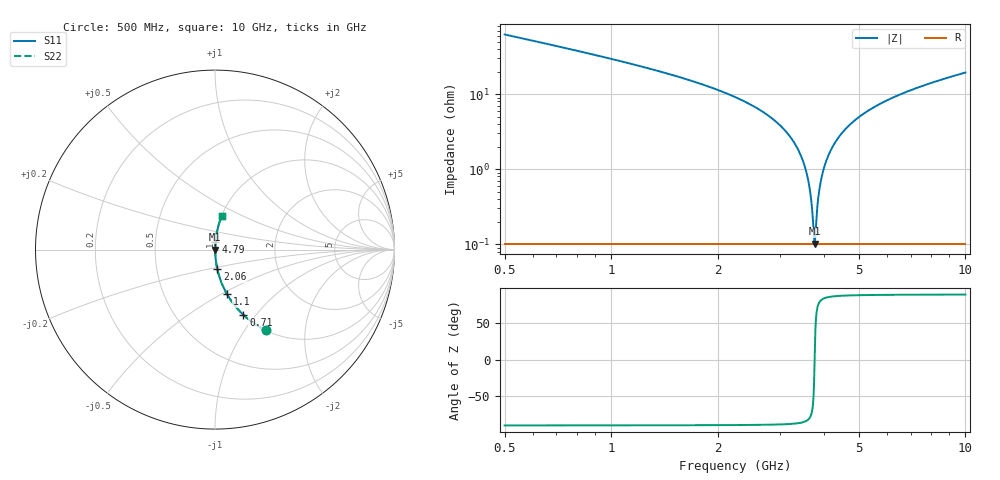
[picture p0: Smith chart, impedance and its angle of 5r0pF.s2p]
! Created Fri Jan 10 15:51:09 2014
# hz S db R 50
! 2 Port Network Data from SP1.SP block
! freq  dbS11  angS11  dbS21  angS21  dbS12  angS12  dbS22  angS22
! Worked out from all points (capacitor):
!   951 points, 500 MHz to 10 GHz, reference 50 ohm
!   read as one part in series: C = 5 pF near 540 MHz
!   lowest |Z| = 101 mohm at 3.75 GHz (marker M1)
!   series resonance near 3.752 GHz, so ESL is about 360 pH
!   S11 on the Smith chart (normalised r, x): 500 MHz: 1.00, -1.25; 710 MHz: 1.00, -0.86; 1.1 GHz: 1.00, -0.53; 2.06 GHz: 1.00, -0.22; 4.79 GHz: 1.00, +0.08; 10 GHz: 1.00, +0.39
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5e8  -5.52 -57.9  -1.44 32.0  -1.44 32.0  -5.52 -57.9
7.1e8  -8.04 -66.5  -0.75 23.4  -0.75 23.4  -8.04 -66.5
1.1e9  -11.85 -75.0  -0.30 14.8  -0.30 14.8  -11.85 -75.0
2.06e9  -19.40 -83.3  -0.06 6.2  -0.06 6.2  -19.40 -83.3
2.09e9  -19.63 -83.5  -0.06 6.0  -0.06 6.0  -19.63 -83.5
2.79e9  -25.87 -85.9  -0.02 2.9  -0.02 2.9  -25.87 -85.9
3.24e9  -32.05 -86.3  -0.01 1.4  -0.01 1.4  -32.05 -86.3
3.52e9  -39.28 -84.1  -0.01 0.6  -0.01 0.6  -39.28 -84.1
3.61e9  -43.59 -80.8  -0.01 0.4  -0.01 0.4  -43.59 -80.8
3.67e9  -48.24 -74.7  -0.01 0.2  -0.01 0.2  -48.24 -74.7
3.72e9  -55.08 -55.0  -0.01 0.1  -0.01 0.1  -55.08 -55.0
3.75e9  -59.89 -4.7  -0.01 0.0  -0.01 0.0  -59.89 -4.7
3.78e9  -55.81 51.4  -0.01 -0.1  -0.01 -0.1  -55.81 51.4
3.84e9  -47.82 75.4  -0.01 -0.2  -0.01 -0.2  -47.82 75.4
3.89e9  -44.13 80.3  -0.01 -0.4  -0.01 -0.4  -44.13 80.3
4.05e9  -37.71 84.8  -0.01 -0.7  -0.01 -0.7  -37.71 84.8
4.34e9  -32.12 86.2  -0.01 -1.4  -0.01 -1.4  -32.12 86.2
4.79e9  -27.58 86.2  -0.02 -2.4  -0.02 -2.4  -27.58 86.2
5.25e9  -24.74 85.7  -0.02 -3.3  -0.02 -3.3  -24.74 85.7
6.84e9  -19.38 83.3  -0.06 -6.2  -0.06 -6.2  -19.38 83.3
8.42e9  -16.44 81.0  -0.11 -8.7  -0.11 -8.7  -16.44 81.0
1e10  -14.40 78.7  -0.17 -11.0  -0.17 -11.0  -14.40 78.7
